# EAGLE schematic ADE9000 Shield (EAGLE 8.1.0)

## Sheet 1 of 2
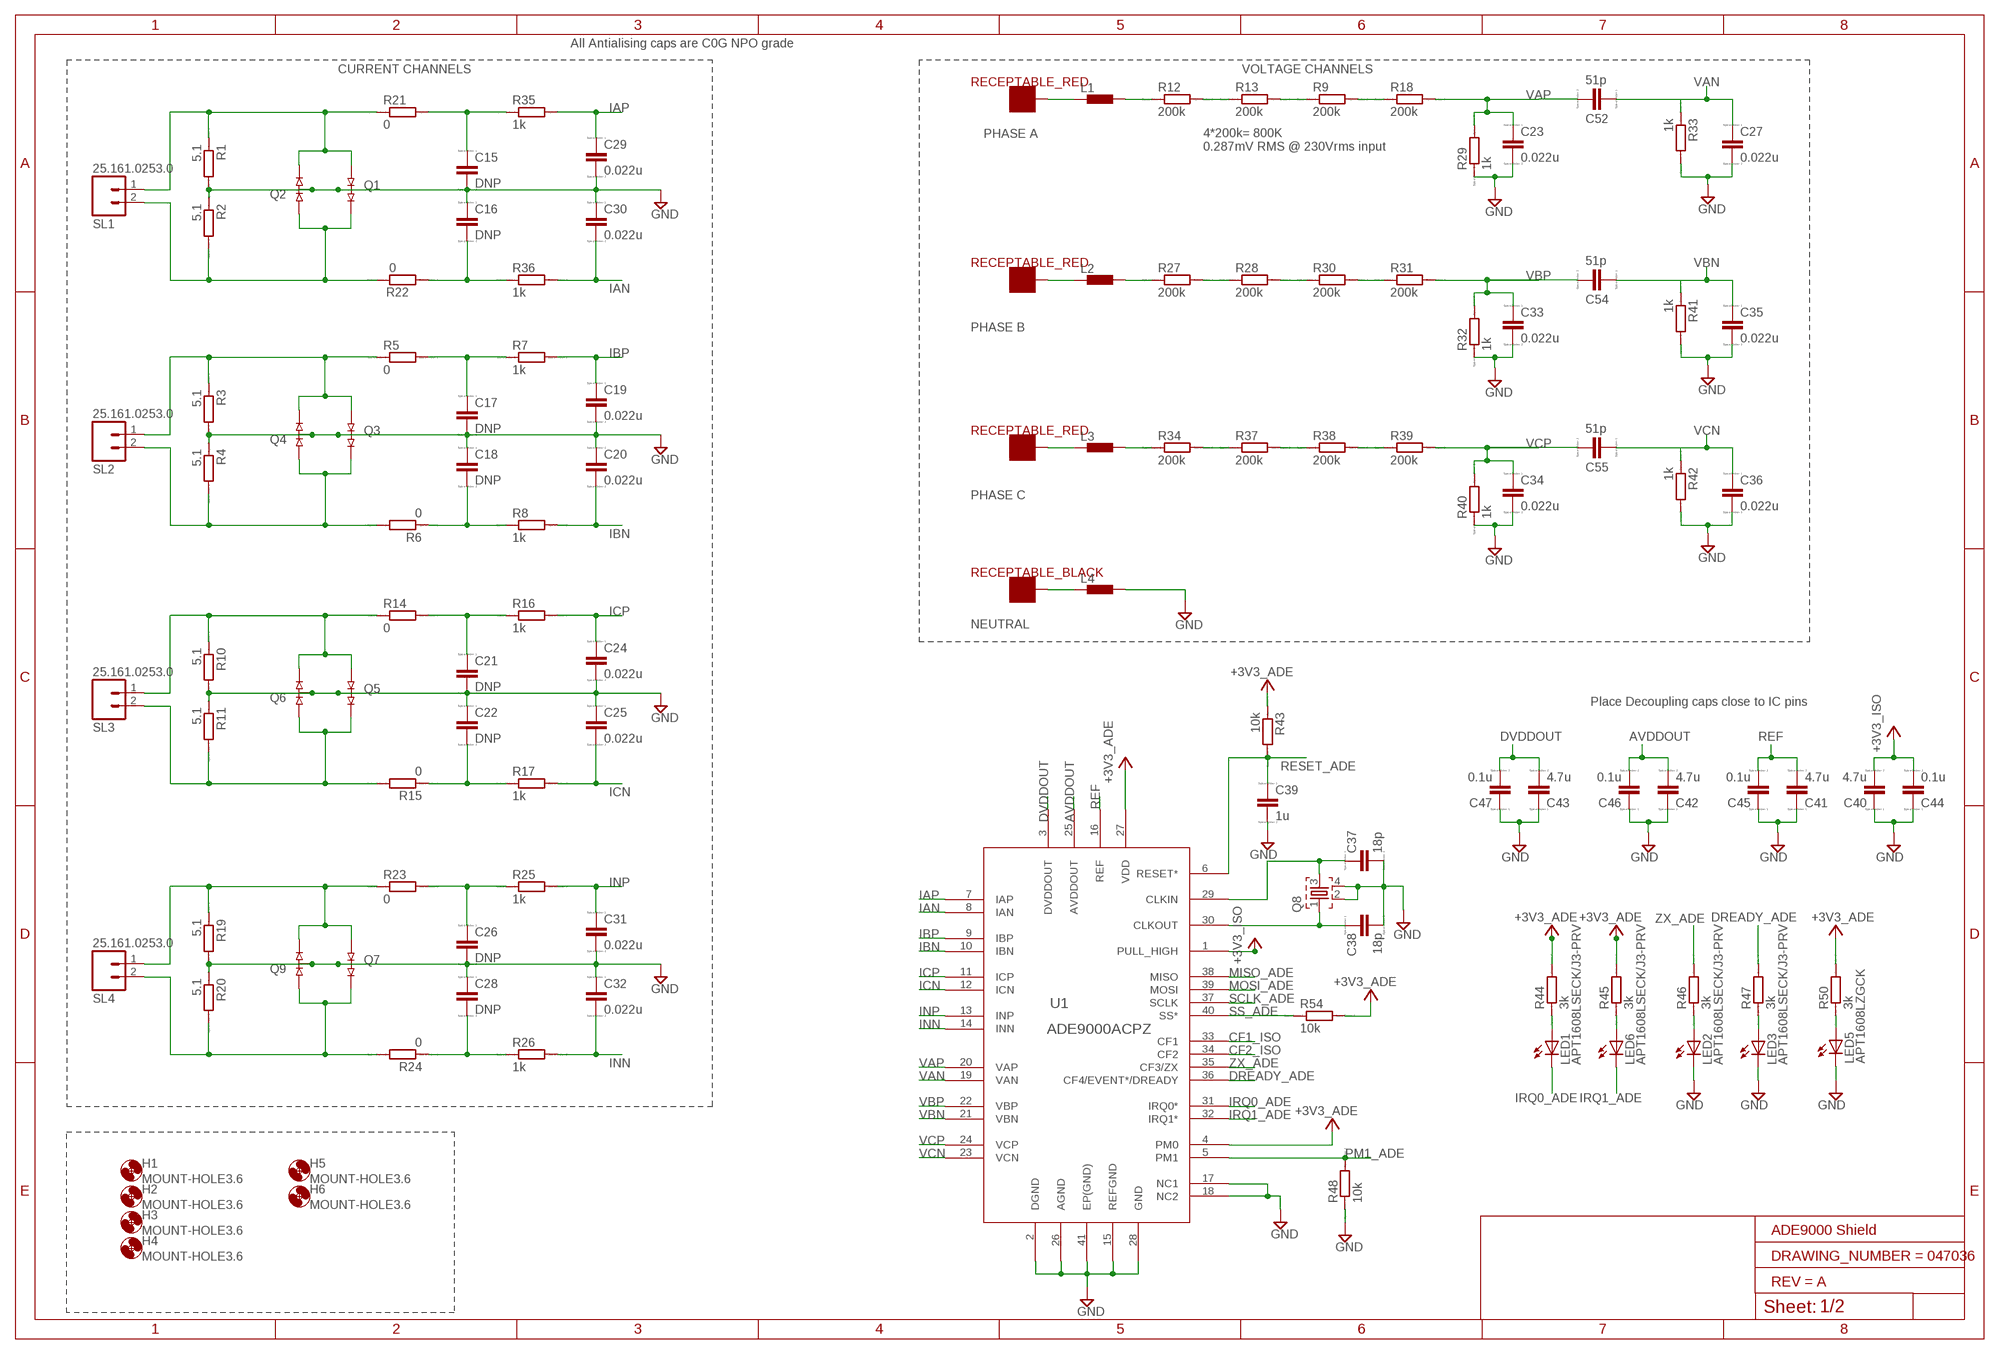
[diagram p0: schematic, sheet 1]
FRAME1 (A3L-LOC): DRAWING_NUMBER: 047036; REV: A

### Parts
C15  DNP  C  [C0805]
C16  DNP  C  [C0805]
C17  DNP  C  [C0805]
C18  DNP  C  [C0805]
C19  0.022u  C  [C0805]
C20  0.022u  C  [C0805]
C21  DNP  C  [C0805]
C22  DNP  C  [C0805]
C23  0.022u  C  [C0805]
C24  0.022u  C  [C0805]
C25  0.022u  C  [C0805]
C26  DNP  C  [C0805]
C27  0.022u  C  [C0805]
C28  DNP  C  [C0805]
C29  0.022u  C  [C0805]
C30  0.022u  C  [C0805]
C31  0.022u  C  [C0805]
C32  0.022u  C  [C0805]
C33  0.022u  C  [C0805]
C34  0.022u  C  [C0805]
C35  0.022u  C  [C0805]
C36  0.022u  C  [C0805]
C37  18p  CC0402  [C0402]
C38  18p  CC0402  [C0402]
C39  1u  CC0603  [C0603]
C40  4.7u  C  [C0805]
C41  4.7u  CC0603  [C0603]
C42  4.7u  CC0603  [C0603]
C43  4.7u  CC0603  [C0603]
C44  0.1u  CC0603  [C0603]
C45  0.1u  CC0603  [C0603]
C46  0.1u  CC0603  [C0603]
C47  0.1u  CC0603  [C0603]
C52  51p  CC0402  [C0402]
C54  51p  CC0402  [C0402]
C55  51p  CC0402  [C0402]
H1  MOUNT-HOLE3.6  [3,6]
H2  MOUNT-HOLE3.6  [3,6]
H3  MOUNT-HOLE3.6  [3,6]
H4  MOUNT-HOLE3.6  [3,6]
H5  MOUNT-HOLE3.6  [3,6]
H6  MOUNT-HOLE3.6  [3,6]
J5  23.3200-22  VOLTAGE_SOCKET_4MM_RED  [SLB4-I/90]
J6  23.3200-22  VOLTAGE_SOCKET_4MM_RED  [SLB4-I/90]
J7  23.3200-22  VOLTAGE_SOCKET_4MM_RED  [SLB4-I/90]
J8  23.3200-21  VOLTAGE_SOCKET_4MM_BLACK  [SLB4-I/90]
L1  1500  FERRITE_BEAD0805  [M0805]
L2  1500  FERRITE_BEAD0805  [M0805]
L3  1500  FERRITE_BEAD0805  [M0805]
L4  1500  FERRITE_BEAD0805  [M0805]
LED1  APT1608LSECK/J3-PRV  LEDSML0603  [SML0603]
LED2  APT1608LSECK/J3-PRV  LEDSML0603  [SML0603]
LED3  APT1608LSECK/J3-PRV  LEDSML0603  [SML0603]
LED5  APT1608LZGCK  LEDSML0603  [SML0603]
LED6  APT1608LSECK/J3-PRV  LEDSML0603  [SML0603]
Q1  MMBD4148SE  DUAL_DIODE_SOT23-3  [SOT23-3]
Q2  MMBD4148SE  DUAL_DIODE_SOT23-3  [SOT23-3]
Q3  MMBD4148SE  DUAL_DIODE_SOT23-3  [SOT23-3]
Q4  MMBD4148SE  DUAL_DIODE_SOT23-3  [SOT23-3]
Q5  MMBD4148SE  DUAL_DIODE_SOT23-3  [SOT23-3]
Q6  MMBD4148SE  DUAL_DIODE_SOT23-3  [SOT23-3]
Q7  MMBD4148SE  DUAL_DIODE_SOT23-3  [SOT23-3]
Q8  ECS-245.7-12-33Q-JES-TR  CRYSTAL_SMD128  [SMD_4PIN_3.2X2.1]
Q9  MMBD4148SE  DUAL_DIODE_SOT23-3  [SOT23-3]
R1  5.1  R  [R0805]
R2  5.1  R  [R0805]
R3  5.1  R  [R0805]
R4  5.1  R  [R0805]
R5  0  RR0603  [R0603]
R6  0  RR0603  [R0603]
R7  1k  RR0603  [R0603]
R8  1k  RR0603  [R0603]
R9  200k  RR2010  [R2010]
R10  5.1  R  [R0805]
R11  5.1  R  [R0805]
R12  200k  RR2010  [R2010]
R13  200k  RR2010  [R2010]
R14  0  RR0603  [R0603]
R15  0  RR0603  [R0603]
R16  1k  RR0603  [R0603]
R17  1k  RR0603  [R0603]
R18  200k  RR2010  [R2010]
R19  5.1  R  [R0805]
R20  5.1  R  [R0805]
R21  0  RR0603  [R0603]
R22  0  RR0603  [R0603]
R23  0  RR0603  [R0603]
R24  0  RR0603  [R0603]
R25  1k  RR0603  [R0603]
R26  1k  RR0603  [R0603]
R27  200k  RR2010  [R2010]
R28  200k  RR2010  [R2010]
R29  1k  RR0603  [R0603]
R30  200k  RR2010  [R2010]
R31  200k  RR2010  [R2010]
R32  1k  RR0603  [R0603]
R33  1k  RR0603  [R0603]
R34  200k  RR2010  [R2010]
R35  1k  RR0603  [R0603]
R36  1k  RR0603  [R0603]
R37  200k  RR2010  [R2010]
R38  200k  RR2010  [R2010]
R39  200k  RR2010  [R2010]
R40  1k  RR0603  [R0603]
R41  1k  RR0603  [R0603]
R42  1k  RR0603  [R0603]
R43  10k  RR0603  [R0603]
R44  3k  RR0603  [R0603]
R45  3k  RR0603  [R0603]
R46  3k  RR0603  [R0603]
R47  3k  RR0603  [R0603]
R48  10k  RR0603  [R0603]
R50  3k  RR0603  [R0603]
R54  10k  RR0603  [R0603]
SL1  25.161.0253.0  M02  [02P]
SL2  25.161.0253.0  M02  [02P]
SL3  25.161.0253.0  M02  [02P]
SL4  25.161.0253.0  M02  [02P]
U1  ADE9000ACPZ  [CP_40_7]

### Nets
+3V3: C40.2 C44.2 R43.1 R44.2 R45.2 R50.2 R54.2 U1.1(PULL_HIGH) U1.4(PM0) U1.27(VDD) ; supply symbol labelled +3V3_ADE, +3V3_ISO ; also sheet 2
AVDDOUT: C42.2 C46.2 U1.25(AVDDOUT)
CF1_ISO: U1.33(CF1)
CF2_ISO: U1.34(CF2)
DREADY_ADE: R47.2 U1.36(CF4/EVENT*/DREADY) ; also sheet 2
DVDDOUT: C43.2 C47.2 U1.3(DVDDOUT)
GND: C15.2 C16.1 C17.2 C18.1 C19.2 C20.1 C21.2 C22.1 C23.2 C24.2 C25.1 C26.2 C27.2 C28.1 C29.2 C30.1 C31.2 C32.1 C33.2 C34.2 C35.2 C36.2 C37.2 C38.2 C39.2 C40.1 C41.1 C42.1 C43.1 C44.1 C45.1 C46.1 C47.1 L4.2 LED2.C LED3.C LED5.C Q1.3 Q2.3 Q3.3 Q4.3 Q5.3 Q6.3 Q7.3 Q8.2 Q8.4 Q9.3 R1.2 R2.1 R3.2 R4.1 R10.2 R11.1 R19.2 R20.1 R29.1 R32.1 R33.2 R40.1 R41.2 R42.2 R48.1 U1.2(DGND) U1.15(REFGND) U1.17(NC1) U1.18(NC2) U1.26(AGND) U1.28(GND) U1.41(EP(GND)) ; also sheet 2
IAN: C30.2 R36.2 U1.8(IAN)
IAP: C29.1 R35.2 U1.7(IAP)
IBN: C20.2 R8.2 U1.10(IBN)
IBP: C19.1 R7.2 U1.9(IBP)
ICN: C25.2 R17.2 U1.12(ICN)
ICP: C24.1 R16.2 U1.11(ICP)
INN: C32.2 R26.2 U1.14(INN)
INP: C31.1 R25.2 U1.13(INP)
IRQ0_ADE: LED1.C U1.31(IRQ0*) ; also sheet 2
IRQ1_ADE: LED6.C U1.32(IRQ1*) ; also sheet 2
MISO_ADE: U1.38(MISO) ; also sheet 2
MOSI_ADE: U1.39(MOSI) ; also sheet 2
N$1: C37.1 Q8.3 U1.29(CLKIN)
N$2: C38.1 Q8.1 U1.30(CLKOUT)
N$3: Q3.1 Q4.2 R3.1 R5.1 SL2.1
N$4: Q3.2 Q4.1 R4.2 R6.2 SL2.2
N$6: C18.2 R6.1 R8.1
N$7: Q1.1 Q2.2 R1.1 R21.1 SL1.1
N$9: C17.1 R5.2 R7.1
N$11: Q5.1 Q6.2 R10.1 R14.1 SL3.1
N$13: Q5.2 Q6.1 R11.2 R15.2 SL3.2
N$14: C16.2 R22.1 R36.1
N$15: J8.P$1 L4.1
N$17: C22.2 R15.1 R17.1
N$18: C21.1 R14.2 R16.1
N$19: LED2.A R46.1
N$21: Q7.1 Q9.2 R19.1 R23.1 SL4.1
N$22: Q7.2 Q9.1 R20.2 R24.2 SL4.2
N$24: C28.2 R24.1 R26.1
N$25: C26.1 R23.2 R25.1
N$27: LED1.A R44.1
N$28: LED6.A R45.1
N$29: LED3.A R47.1
N$32: L2.2 R27.1
N$33: R27.2 R28.1
N$34: R28.2 R30.1
N$35: L1.2 R12.1
N$36: R12.2 R13.1
N$37: R9.1 R13.2
N$38: R9.2 R18.1
N$40: Q1.2 Q2.1 R2.2 R22.2 SL1.2
N$41: C15.1 R21.2 R35.1
N$42: R30.2 R31.1
N$45: L3.2 R34.1
N$46: R34.2 R37.1
N$47: R37.2 R38.1
N$48: R38.2 R39.1
N$50: LED5.A R50.1
N$67: J5.P$1 L1.1
N$68: J6.P$1 L2.1
N$69: J7.P$1 L3.1
PM1_ADE: R48.2 U1.5(PM1) ; also sheet 2
REF: C41.2 C45.2 U1.16(REF)
RESET_ADE: C39.1 R43.2 U1.6(RESET*) ; also sheet 2
SCLK_ADE: U1.37(SCLK) ; also sheet 2
SS_ADE: R54.1 U1.40(SS*) ; also sheet 2
VAN: C27.1 C52.1 R33.1 U1.19(VAN)
VAP: C23.1 C52.2 R18.2 R29.2 U1.20(VAP)
VBN: C35.1 C54.1 R41.1 U1.21(VBN)
VBP: C33.1 C54.2 R31.2 R32.2 U1.22(VBP)
VCN: C36.1 C55.1 R42.1 U1.23(VCN)
VCP: C34.1 C55.2 R39.2 R40.2 U1.24(VCP)
ZX_ADE: R46.2 U1.35(CF3/ZX) ; also sheet 2

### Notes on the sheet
- All Antialising caps are C0G NPO grade
- CURRENT CHANNELS | VOLTAGE CHANNELS
- PHASE A
- 4*200k= 800K
  0.287mV RMS @ 230Vrms input
- PHASE B
- PHASE C
- NEUTRAL
- Place Decoupling caps close to IC pins

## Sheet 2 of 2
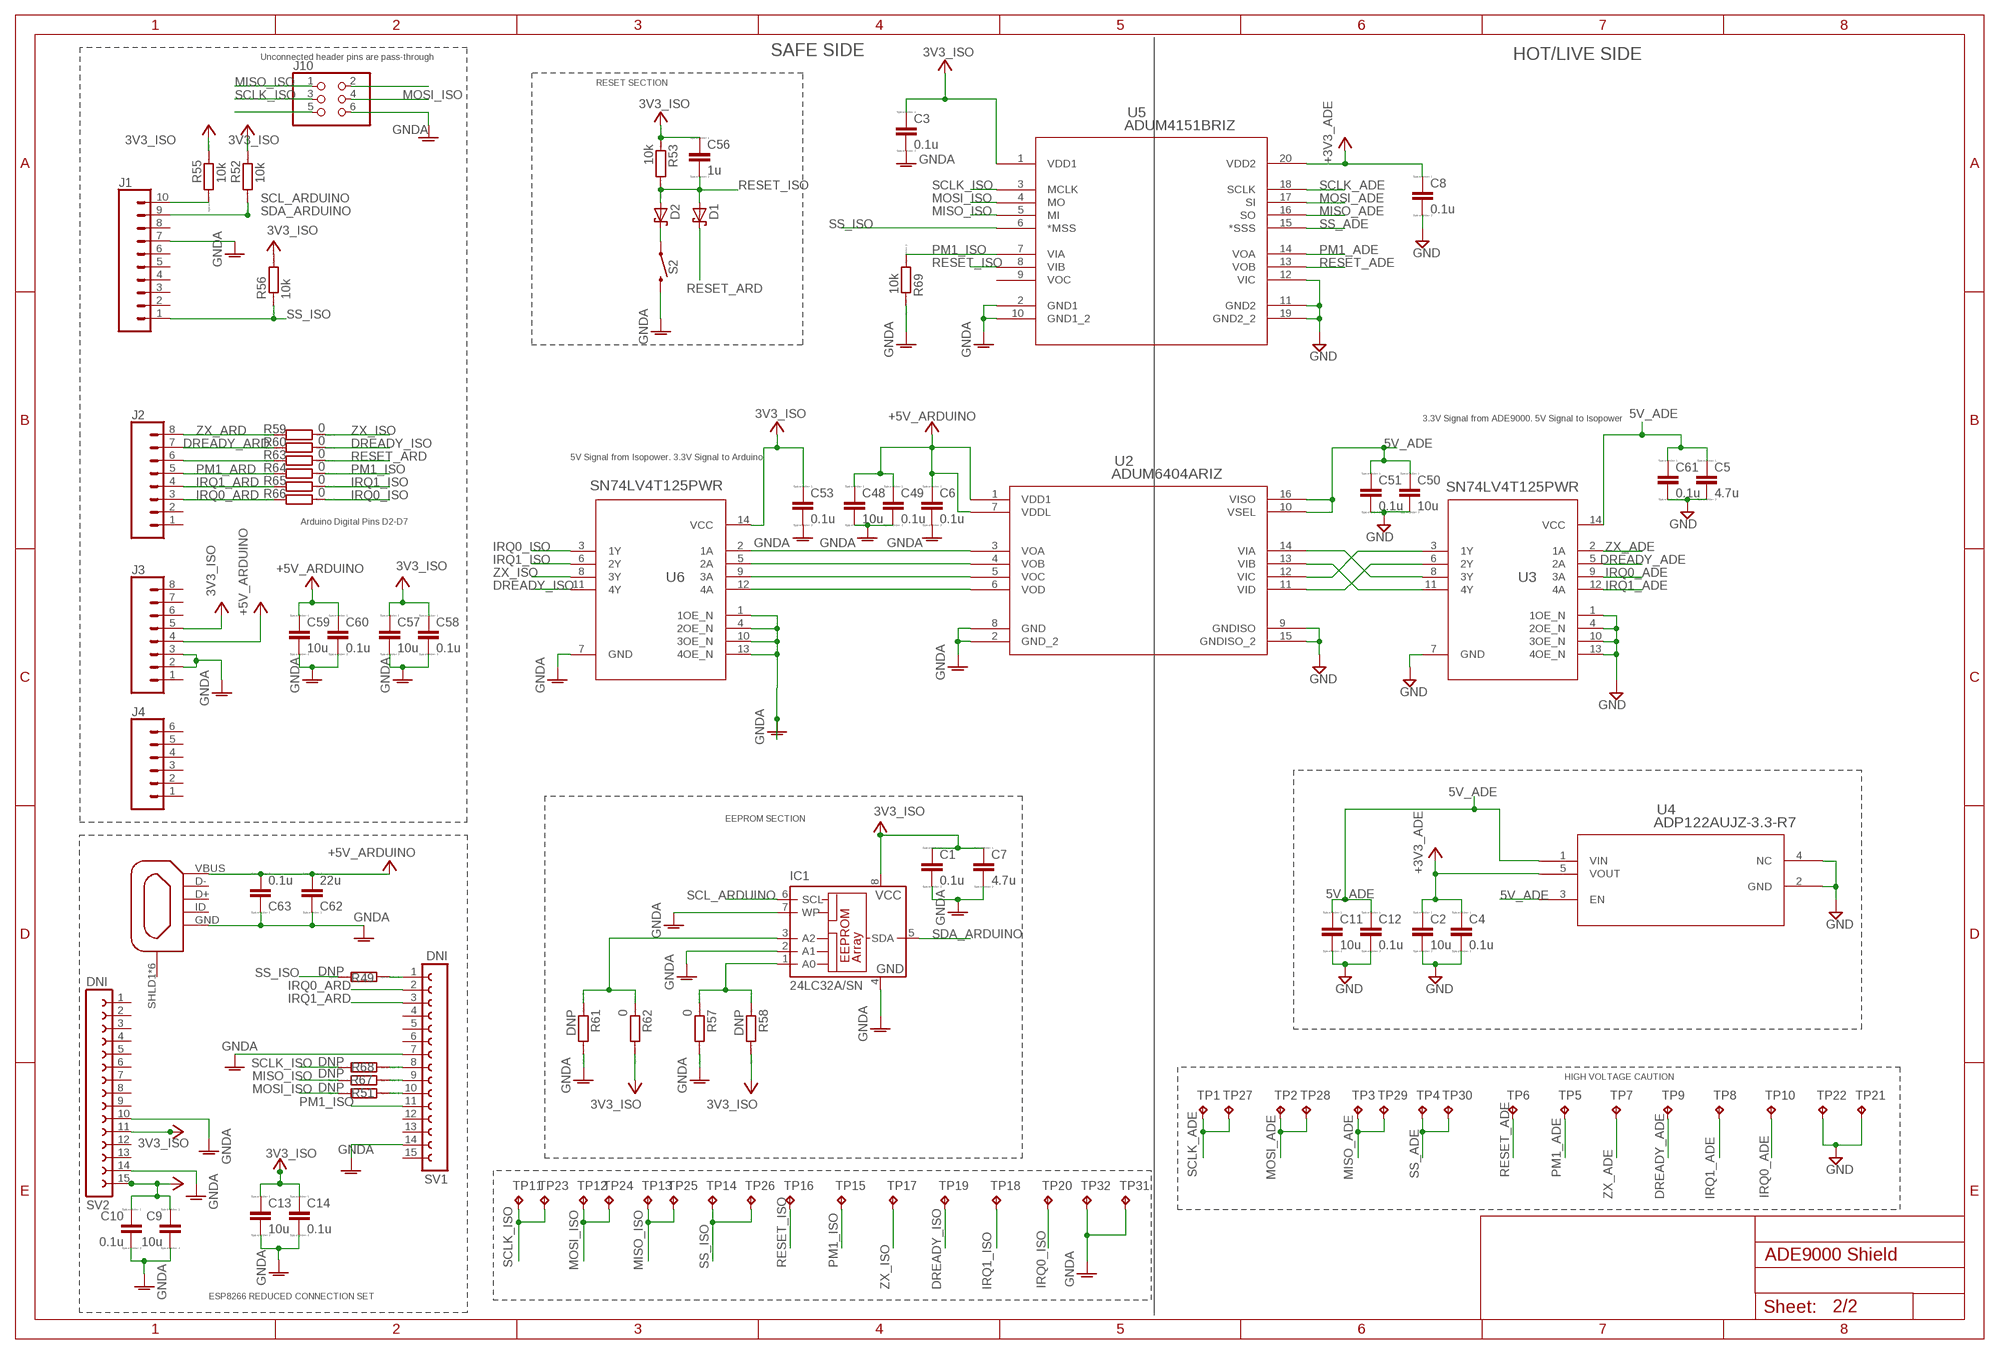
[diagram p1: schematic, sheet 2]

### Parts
C1  0.1u  CC0603  [C0603]
C2  10u  C  [C0805]
C3  0.1u  CC0603  [C0603]
C4  0.1u  CC0603  [C0603]
C5  4.7u  C  [C0805]
C6  0.1u  CC0603  [C0603]
C7  4.7u  C  [C0805]
C8  0.1u  CC0603  [C0603]
C9  10u  C  [C0805]
C10  0.1u  CC0603  [C0603]
C11  10u  C  [C0805]
C12  0.1u  CC0603  [C0603]
C13  10u  C  [C0805]
C14  0.1u  CC0603  [C0603]
C48  10u  C  [C0805]
C49  0.1u  CC0603  [C0603]
C50  10u  C  [C0805]
C51  0.1u  CC0603  [C0603]
C53  0.1u  CC0603  [C0603]
C56  1u  CC0603  [C0603]
C57  10u  C  [C0805]
C58  0.1u  CC0603  [C0603]
C59  10u  C  [C0805]
C60  0.1u  CC0603  [C0603]
C61  0.1u  CC0603  [C0603]
C62  22u  C  [C0805]
C63  0.1u  CC0603  [C0603]
D1  BAT54WS  BAT60J  [SOD323_ST]
D2  BAT54WS  BAT60J  [SOD323_ST]
IC1  24LC32A/SN  24LC32ASN  [SO-08]
J1  CONN_10NO_SILK_PTH_FEMALE  [1X10_NO_SILK]
J2  CONN_08NO_SILK_FEMALE_PTH  [1X08_NO_SILK]
J3  CONN_08NO_SILK_FEMALE_PTH  [1X08_NO_SILK]
J4  CONN_06NO_SILK_FEMALE_PTH  [1X06_NO_SILK]
J9  ZX62-AB-5PA(31)  USB_MICRO  [USB-MICRO-10103594]
J10  ARDUINO_ICSP  [ARDUINO_2X03]
R49  DNP  RR0603  [R0603]
R51  DNP  RR0603  [R0603]
R52  10k  RR0603  [R0603]
R53  10k  RR0603  [R0603]
R55  10k  RR0603  [R0603]
R56  10k  RR0603  [R0603]
R57  0  RR0603  [R0603]
R58  DNP  RR0603  [R0603]
R59  0  RR0603  [R0603]
R60  0  RR0603  [R0603]
R61  DNP  RR0603  [R0603]
R62  0  RR0603  [R0603]
R63  0  RR0603  [R0603]
R64  0  RR0603  [R0603]
R65  0  RR0603  [R0603]
R66  0  RR0603  [R0603]
R67  DNP  RR0603  [R0603]
R68  DNP  RR0603  [R0603]
R69  10k  RR0603  [R0603]
S2  PTS645SM43SMTR92  MOMENTARY-SWITCH-SPST-SMD-6.2MM-TALL  [TACTILE_SWITCH_SMD_6.2MM_TALL]
SV1  DNI  FE15-1  [FE15]
SV2  DNI  FE15-1  [FE15]
TP1  TPTP20SQ  [TP20SQ]
TP2  TPTP20SQ  [TP20SQ]
TP3  TPTP20SQ  [TP20SQ]
TP4  TPTP20SQ  [TP20SQ]
TP5  TPPAD1-17  [P1-17]
TP6  TPPAD1-17  [P1-17]
TP7  TPPAD1-17  [P1-17]
TP8  TPPAD1-17  [P1-17]
TP9  TPPAD1-17  [P1-17]
TP10  TPPAD1-17  [P1-17]
TP11  TPTP20SQ  [TP20SQ]
TP12  TPTP20SQ  [TP20SQ]
TP13  TPTP20SQ  [TP20SQ]
TP14  TPTP20SQ  [TP20SQ]
TP15  TPPAD1-17  [P1-17]
TP16  TPPAD1-17  [P1-17]
TP17  TPPAD1-17  [P1-17]
TP18  TPPAD1-17  [P1-17]
TP19  TPPAD1-17  [P1-17]
TP20  TPPAD1-17  [P1-17]
TP21  TPPAD1-17  [P1-17]
TP22  TPPAD1-17  [P1-17]
TP23  TPTP20SQ  [TP20SQ]
TP24  TPTP20SQ  [TP20SQ]
TP25  TPTP20SQ  [TP20SQ]
TP26  TPTP20SQ  [TP20SQ]
TP27  TPTP20SQ  [TP20SQ]
TP28  TPTP20SQ  [TP20SQ]
TP29  TPTP20SQ  [TP20SQ]
TP30  TPTP20SQ  [TP20SQ]
TP31  TPPAD1-17  [P1-17]
TP32  TPPAD1-17  [P1-17]
U2  ADUM6404ARIZ  [RI_16_1]
U3  SN74LV4T125PWR  [PW0014A_N]
U4  ADP122AUJZ-3.3-R7  [UJ_5]
U5  ADUM4151BRIZ  ADUM4151ARIZ  [RI_20_1]
U6  SN74LV4T125PWR  [PW0014A_N]

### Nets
5V_ADE: C5.1 C11.1 C12.1 C50.1 C51.1 C61.1 U2.10(VSEL) U2.16(VISO) U3.14(VCC) U4.1(VIN) U4.3(EN)
+3V3: C2.1 C4.1 C8.1 U4.5(VOUT) U5.20(VDD2) ; supply symbol labelled +3V3_ADE ; also sheet 1
DREADY_ADE: TP9.TP U3.5(2A) ; also sheet 1
DREADY_ARD: J2.7 R60.2
DREADY_ISO: R60.1 TP19.TP U6.11(4Y)
GND: C2.2 C4.2 C5.2 C8.2 C11.2 C12.2 C50.2 C51.2 C61.2 TP21.TP TP22.TP U2.9(GNDISO) U2.15(GNDISO_2) U3.1(1OE_N) U3.4(2OE_N) U3.7(GND) U3.10(3OE_N) U3.13(4OE_N) U4.2(GND) U4.4(NC) U5.11(GND2) U5.12(VIC) U5.19(GND2_2) ; also sheet 1
GNDA: C1.2 C3.2 C6.2 C7.2 C9.2 C10.2 C13.2 C14.2 C48.2 C49.2 C53.2 C57.2 C58.2 C59.2 C60.2 C62.1 C63.1 IC1.2(A1) IC1.4(GND) IC1.7(WP) J1.7 J3.2 J3.3 J9.GND J10.6 R57.2 R61.2 R69.2 S2.B2 SV1.7 SV1.14 SV2.10 SV2.14 TP31.TP TP32.TP U2.2(GND_2) U2.8(GND) U5.2(GND1) U5.10(GND1_2) U6.1(1OE_N) U6.4(2OE_N) U6.7(GND) U6.10(3OE_N) U6.13(4OE_N)
IRQ0_ADE: TP10.TP U3.9(3A) ; also sheet 1
IRQ0_ARD: J2.3 R66.2 SV1.2
IRQ0_ISO: R66.1 TP20.TP U6.3(1Y)
IRQ1_ADE: TP8.TP U3.12(4A) ; also sheet 1
IRQ1_ARD: J2.4 R65.2 SV1.3
IRQ1_ISO: R65.1 TP18.TP U6.6(2Y)
MISO_ADE: TP3.TP TP29.TP U5.16(SO) ; also sheet 1
MISO_ISO: J10.1 R67.2 TP13.TP TP25.TP U5.5(MI)
MOSI_ADE: TP2.TP TP28.TP U5.17(SI) ; also sheet 1
MOSI_ISO: J10.4 R51.2 TP12.TP TP24.TP U5.4(MO)
N$8: IC1.3(A2) R61.1 R62.1
N$16: J2.6 R63.2
N$23: R49.1 SV1.1
N$30: U2.14(VIA) U3.8(3Y)
N$31: U2.13(VIB) U3.11(4Y)
N$39: D2.C S2.A2
N$44: U2.12(VIC) U3.3(1Y)
N$49: U2.11(VID) U3.6(2Y)
N$51: J10.2
N$52: R68.1 SV1.8
N$53: R67.1 SV1.9
N$55: R51.1 SV1.10
N$57: U2.3(VOA) U6.2(1A)
N$58: U2.4(VOB) U6.5(2A)
N$59: U2.5(VOC) U6.9(3A)
N$60: U2.6(VOD) U6.12(4A)
N$74: J10.5
N$76: IC1.1(A0) R57.1 R58.1
PM1_ADE: TP5.TP U5.14(VOA) ; also sheet 1
PM1_ARD: J2.5 R64.2
PM1_ISO: R64.1 R69.1 SV1.11 TP15.TP U5.7(VIA)
RESET_ADE: TP6.TP U5.13(VOB) ; also sheet 1
RESET_ARD: D1.C R63.1
RESET_ISO: C56.2 D1.A D2.A R53.2 TP16.TP U5.8(VIB)
SCL_ARDUINO: IC1.6(SCL) J1.10 R55.1
SCLK_ADE: TP1.TP TP27.TP U5.18(SCLK) ; also sheet 1
SCLK_ISO: J10.3 R68.2 TP11.TP TP23.TP U5.3(MCLK)
SDA_ARDUINO: IC1.5(SDA) J1.9 R52.1
SS_ADE: TP4.TP TP30.TP U5.15(*SSS) ; also sheet 1
SS_ISO: J1.1 R49.2 R56.1 TP14.TP TP26.TP U5.6(*MSS)
V+: C1.1 C3.1 C7.1 C13.1 C14.1 C53.1 C56.1 C57.1 C58.1 IC1.8(VCC) J3.5 R52.2 R53.1 R55.2 R56.2 R58.2 R62.2 SV2.11 U5.1(VDD1) U6.14(VCC) ; supply symbol labelled 3V3_ISO
VCC: C6.1 C9.1 C10.1 C48.1 C49.1 C59.1 C60.1 C62.2 C63.2 J3.4 J9.VBUS SV2.15 U2.1(VDD1) U2.7(VDDL) ; supply symbol labelled +5V_ARDUINO
ZX_ADE: TP7.TP U3.2(1A) ; also sheet 1
ZX_ARD: J2.8 R59.2
ZX_ISO: R59.1 TP17.TP U6.8(3Y)
Unconnected: J1.2 J1.3 J1.4 J1.5 J1.6 J1.8 J2.1 J2.2 J3.1 J3.6 J3.7 J3.8 J4.1 J4.2 J4.3 J4.4 J4.5 J4.6 J9.D+ J9.D- J9.ID J9.SHLD1(SHLD1*6) J9.SHLD2(SHLD1*6) J9.SHLD3(SHLD1*6) J9.SHLD4(SHLD1*6) J9.SHLD5(SHLD1*6) J9.SHLD6(SHLD1*6) SV1.4 SV1.5 SV1.6 SV1.12 SV1.13 SV1.15 SV2.1 SV2.2 SV2.3 SV2.4 SV2.5 SV2.6 SV2.7 SV2.8 SV2.9 SV2.12 SV2.13 U5.9(VOC)

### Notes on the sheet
- SAFE SIDE
- Unconnected header pins are pass-through | HOT/LIVE SIDE
- RESET SECTION
- 3.3V Signal from ADE9000. 5V Signal to Isopower
- 5V Signal from Isopower. 3.3V Signal to Arduino
- Arduino Digital Pins D2-D7
- EEPROM SECTION
- HIGH VOLTAGE CAUTION
- ESP8266 REDUCED CONNECTION SET

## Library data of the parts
C1-C14 C48-C51 C53 C57-C63 = eagle-ltspice:C: CAPACITOR, European symbol; SPICEMODEL: NONE; SPICEPREFIX: C
C15-C47 C52 C54-C56 = capacitors:C: CAPACITOR, European symbol; SPICEMODEL: NONE; SPICEPREFIX: C
D1 D2 = diode:BAT60J: Schottky barrier diode
H1-H6 = holes:MOUNT-HOLE: MOUNTING HOLE with drill center marker
IC1 = microchip:24*: Serial EEPROM I2C; MF: MICROCHIP; MPN: 24LC32A/SN; OC_FARNELL: 9758003; OC_NEWARK: 33C2976
J1 = SparkFun-Connectors:CONN_10: Multi connection point. Often used as Generic Header-pin footprint for 0.1 inch spaced/style header connections On any of the 0.1 inch spaced packages, you can populate with these: Break Away Headers - Straight (PRT-00116) Break Away Male Headers - Right Angle (PRT-00553) Female Headers (PRT-00115)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; PROD_ID: CONN-11563
J2 J3 = SparkFun-Connectors:CONN_08: Multi connection point. Often used as Generic Header-pin footprint for 0.1 inch spaced/style header connections On any of the 0.1 inch spaced packages, you can populate with these: Break Away Headers - Straight (PRT-00116) Break Away Male Headers - Right Angle (PRT-00553) Female Headers (PRT-00115)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; PROD_ID: CONN-08438
J4 = SparkFun-Connectors:CONN_06: Multi connection point. Often used as Generic Header-pin footprint for 0.1 inch spaced/style header connections On any of the 0.1 inch spaced packages, you can populate with these: Break Away Headers - Straight (PRT-00116) Break Away Male Headers - Right Angle (PRT-00553) Female Headers (PRT-00115)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; PROD_ID: CONN-08437
J5-J7 = Connectors:VOLTAGE_SOCKET_4MM_RED; NEWARK: 15J4893
J8 = Connectors:VOLTAGE_SOCKET_4MM_BLACK; NEWARK: 98K7138
J9 = Connectors:USB_MICRO; MANUFACTURER: Hirose Electric; MFRPART#: ZX62-AB-5PA(31)
J10 = Connectors:ARDUINO_ICSP: PIN HEADER
L1-L4 = Inductors:FERRITE_BEAD; DIGIKEY: 490-1048-1-ND
LED1-LED3 LED6 = DIODE_LED:LED: LED; PARTNO: APT1608LSECK/J3-PRV
LED5 = DIODE_LED:LED: LED; PARTNO: APT1608LZGCK
Q1-Q7 Q9 = DIODE_LED:DUAL_DIODE; DIGIKEY: MMBD4148SECT-ND
Q8 = Crystals:CRYSTAL_SMD; DIGIKEY: XC2178CT-ND
R1 = eagle-ltspice:R: RESISTOR, European symbol; DESCRIPTION: RES, 5.1, 0W1, 0%1, 0805-SMT, ROHS; MANUFACTURER: TE Connectivity Passive Product; MFR_PART_NO_#: CPF0805B5R1E1; SPICEMODEL: NONE; SPICEPREFIX: R
R2-R69 = eagle-ltspice:R: RESISTOR, European symbol; SPICEMODEL: NONE; SPICEPREFIX: R
S2 = SparkFun-Switches:MOMENTARY-SWITCH-SPST: Momentary Switch (Pushbutton) - SPST; PROD_ID: SWCH-11966; SF_SKU: COM-12992
SL1-SL4 = GEEC_LibrariesCon_GEEC_Voltage:M02: AMP QUICK CONNECTOR; OC_FARNELL: unknown; OC_NEWARK: unknown
SV1 SV2 = con-lsta:FE15-1: FEMALE HEADER; OC_FARNELL: unknown; OC_NEWARK: unknown
TP1-TP32 = testpad:TP: Test pad
U1 = IC:ADE9000ACPZ; DIGIKEY: ADE9000ACPZ-RLCT-ND
U2 = IC:ADUM6404ARIZ
U3 U6 = IC:SN74LV4T125PWR; COMPTYPE: IC; MANUFACTURER: Texas Instruments; MOUNTTYPE: SMT; PACKAGEREFERENCE: PW0014A; PARTNUMBER: SN74LV4T125PWR; PIN_COUNT: 14; REFDES: RefDes; ROHS: Y; TYPE: TYPE; VALUE: Value
U4 = IC:ADP122AUJZ-3.3-R7
U5 = IC:ADUM4151ARIZ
